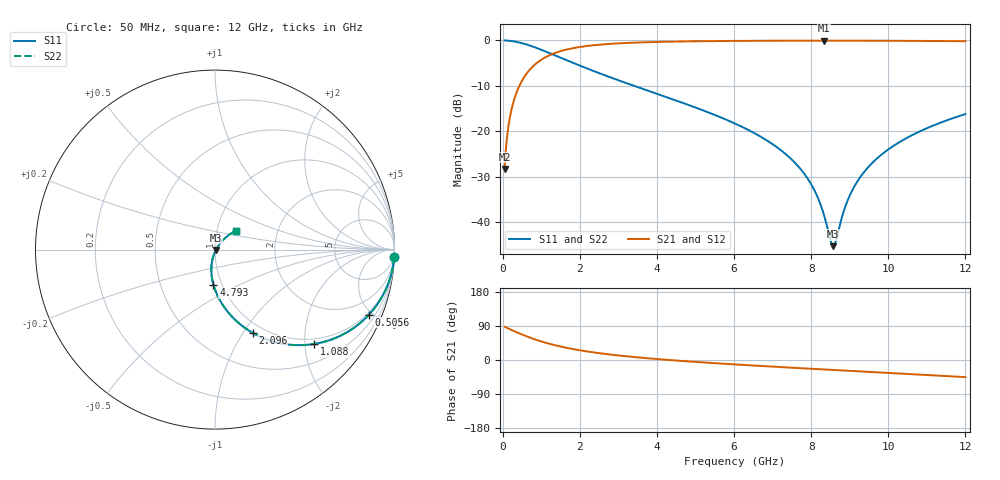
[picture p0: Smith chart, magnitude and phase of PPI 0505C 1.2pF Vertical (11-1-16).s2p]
# GHz S MA R 50
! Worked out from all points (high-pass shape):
!   1601 points, 50 MHz to 12 GHz, reference 50 ohm
!   highest |S21| = -0.05 dB at 8.325 GHz (marker M1); lowest = -28.3 dB at 50 MHz (marker M2)
!   |S21| within 3 dB of the highest: 1.272 GHz to end of sweep
!   lowest |S11| = -45.3 dB at 8.572 GHz (marker M3), VSWR 1.01, Z = 50.5 - j0.254 ohm
!   |S11| at or under -10 dB: 3.406 GHz to end of sweep
!   |S22| runs from -45.3 to 0.0 dB; largest |S21 - S12| = 0
!   S11 on the Smith chart (normalised r, x): 50 MHz: 1, -49; 505.6 MHz: 0.88, -4.80; 1.088 GHz: 0.88, -2.21; 2.096 GHz: 0.88, -1.10; 4.793 GHz: 0.91, -0.37; 12 GHz: 1.23, +0.26
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0.05  0.9993 -2.4  0.03837 87.6  0.03837 87.6  0.9993 -2.4
0.1470937  0.9937 -6.9  0.1123 83.1  0.1123 83.1  0.9937 -6.9
0.22925  0.9848 -10.7  0.1735 79.3  0.1735 79.3  0.9848 -10.7
0.5055937  0.9316 -22.8  0.3627 67.1  0.3627 67.1  0.9316 -22.8
1.088156  0.7627 -43.6  0.6452 46.3  0.6452 46.3  0.7627 -43.6
2.044156  0.5192 -64.8  0.8521 24.9  0.8521 24.9  0.5192 -64.8
2.096437  0.5087 -65.7  0.8584 24.0  0.8584 24.0  0.5087 -65.7
2.925469  0.374 -76.7  0.9243 12.8  0.9243 12.8  0.374 -76.7
4.038312  0.2549 -87.0  0.9632 2.2  0.9632 2.2  0.2549 -87.0
4.792656  0.1965 -92.4  0.9764 -3.6  0.9764 -3.6  0.1965 -92.4
6.025  0.1214 -99.6  0.9879 -11.7  0.9879 -11.7  0.1214 -99.6
7.264812  0.05944 -104.3  0.9929 -19.0  0.9929 -19.0  0.05944 -104.3
8.019156  0.02523 -101.4  0.994 -23.2  0.994 -23.2  0.02523 -101.4
8.325375  0.01224 -89.2  0.9941 -24.9  0.9941 -24.9  0.01224 -89.2
8.504625  0.00621 -55.8  0.9941 -25.9  0.9941 -25.9  0.00621 -55.8
8.571844  0.005417 -27.6  0.994 -26.3  0.994 -26.3  0.005417 -27.6
8.639062  0.00614 0.9  0.994 -26.7  0.994 -26.7  0.00614 0.9
8.907937  0.01568 41.1  0.9938 -28.1  0.9938 -28.1  0.01568 41.1
9.139469  0.02546 47.7  0.9934 -29.4  0.9934 -29.4  0.02546 47.7
9.512906  0.04162 50.5  0.9927 -31.4  0.9927 -31.4  0.04162 50.5
10.01331  0.06357 50.3  0.9913 -34.2  0.9913 -34.2  0.06357 50.3
12  0.1546 42.2  0.9801 -45.1  0.9801 -45.1  0.1546 42.2
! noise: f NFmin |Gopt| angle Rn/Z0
0.05  0.001054  0.9646  1.601  0.006732
1.372  0.00584  0.7686  6.181  0.005124
2.701  0.009211  0.7174  9.865  0.006398
4.031  0.01219  0.6873  13.64  0.007472
5.36  0.01501  0.6672  17.41  0.008465
6.682  0.01773  0.6537  21.11  0.009435
8.012  0.02047  0.6448  24.78  0.01044
9.341  0.02327  0.6398  28.37  0.0115
10.67  0.02617  0.638  31.89  0.01265
12  0.02922  0.6392  35.33  0.01394
